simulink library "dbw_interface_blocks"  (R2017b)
settings: Solver=ode1  StartTime=0.0  StopTime=Inf  FixedStep=0.001  RelTol=1e-3  EnableMultiTasking=on
PostLoadFcn:
  | , if any(exist('dsrtsu_mdlpostloadfcn', 'file') == [2, 3, 6]), try dsrtsu_mdlpostloadfcn('Execute', bdroot); catch fprintf('Error in PostLoadFcn (dsrtsu_mdlpostloadfcn) for model "%s":\n %s\n', bdroot, lasterr); end, end,
libraries: rtican x9

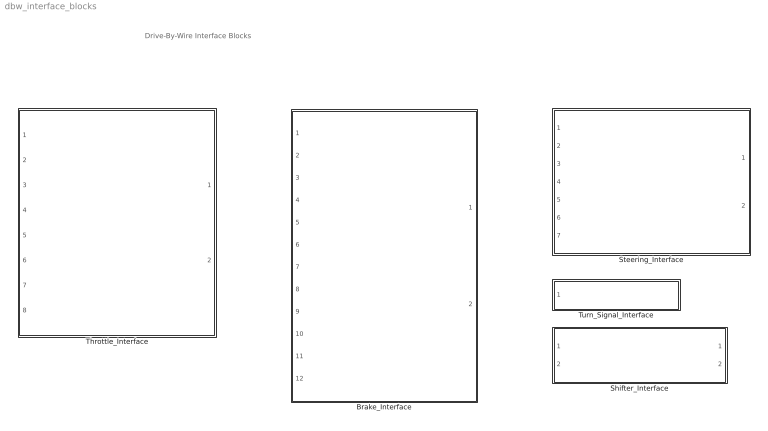
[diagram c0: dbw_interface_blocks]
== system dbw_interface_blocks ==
  note: Drive-By-Wire Interface Blocks
  Brake_Interface : Subsystem
  Shifter_Interface : Subsystem
  Steering_Interface : Subsystem
  Throttle_Interface : Subsystem
  Turn_Signal_Interface : Subsystem

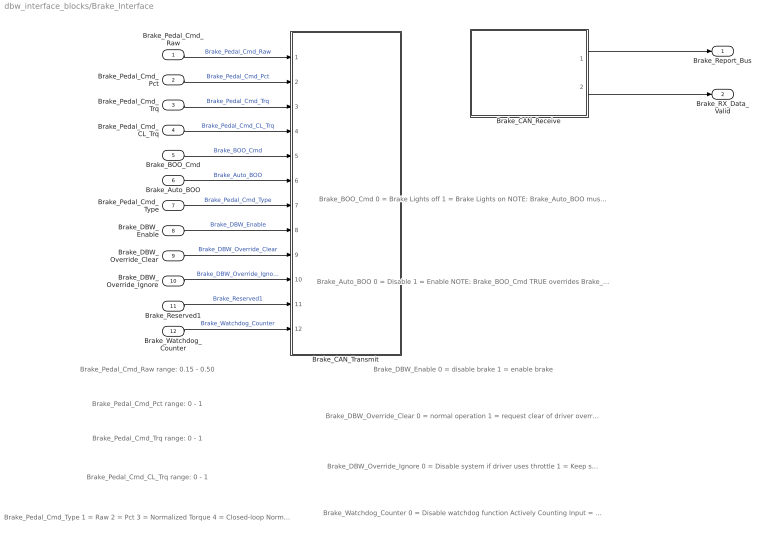
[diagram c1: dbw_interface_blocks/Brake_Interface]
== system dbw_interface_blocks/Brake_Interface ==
  note: Brake_Watchdog_Counter 0 = Disable watchdog function Actively Counting Input = Enable watchdog function
  note: Brake_DBW_Override_Ignore 0 = Disable system if driver uses throttle 1 = Keep system enabled if driver uses throttle
  note: Brake_DBW_Override_Clear 0 = normal operation 1 = request clear of driver override
  note: Brake_BOO_Cmd 0 = Brake Lights off 1 = Brake Lights on NOTE: Brake_Auto_BOO must be set to FALSE for user to have full control over Brake Lights On/Off.
  note: Brake_Pedal_Cmd_Raw range: 0.15 - 0.50
  note: Brake_DBW_Enable 0 = disable brake 1 = enable brake
  note: Brake_Pedal_Cmd_Pct range: 0 - 1
  note: Brake_Pedal_Cmd_Type 1 = Raw 2 = Pct 3 = Normalized Torque 4 = Closed-loop Normalized Torque
  note: Brake_Pedal_Cmd_Trq range: 0 - 1
  note: Brake_Pedal_Cmd_CL_Trq range: 0 - 1
  note: Brake_Auto_BOO 0 = Disable 1 = Enable NOTE: Brake_BOO_Cmd TRUE overrides Brake_Auto_BOO .
  Brake_Pedal_Cmd_Raw : Inport
  Brake_Pedal_Cmd_Pct : Inport  Port=2
  Brake_Pedal_Cmd_Trq : Inport  Port=3
  Brake_Pedal_Cmd_CL_Trq : Inport  Port=4
  Brake_BOO_Cmd : Inport  Port=5
  Brake_Auto_BOO : Inport  Port=6
  Brake_Pedal_Cmd_Type : Inport  Port=7
  Brake_DBW_Enable : Inport  Port=8
  Brake_DBW_Override_Clear : Inport  Port=9
  Brake_DBW_Override_Ignore : Inport  Port=10
  Brake_Reserved1 : Inport  Port=11
  Brake_Watchdog_Counter : Inport  Port=12
  Brake_CAN_Receive : Subsystem
  Brake_CAN_Transmit : Subsystem
  Brake_Report_Bus : Outport
  Brake_RX_Data_Valid : Outport  Port=2
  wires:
  Brake_Watchdog_Counter/1 -> Brake_CAN_Transmit/12(Brake_Watchdog_Counter)  "Brake_Watchdog_Counter"
  Brake_DBW_Override_Ignore/1 -> Brake_CAN_Transmit/10(Brake_DBW_Override_Ignore)  "Brake_DBW_Override_Ignore"
  Brake_CAN_Receive/1(Brake_Report_Bus) -> Brake_Report_Bus/1
  Brake_DBW_Override_Clear/1 -> Brake_CAN_Transmit/9(Brake_DBW_Override_Clear)  "Brake_DBW_Override_Clear"
  Brake_CAN_Receive/2(Brake_RX_Data_Valid) -> Brake_RX_Data_Valid/1
  Brake_BOO_Cmd/1 -> Brake_CAN_Transmit/5(Brake_BOO_Cmd)  "Brake_BOO_Cmd"
  Brake_DBW_Enable/1 -> Brake_CAN_Transmit/8(Brake_DBW_Enable)  "Brake_DBW_Enable"
  Brake_Reserved1/1 -> Brake_CAN_Transmit/11(Brake_Reserved1)  "Brake_Reserved1"
  Brake_Auto_BOO/1 -> Brake_CAN_Transmit/6(Brake_Auto_BOO)  "Brake_Auto_BOO"
  Brake_Pedal_Cmd_Type/1 -> Brake_CAN_Transmit/7(Brake_Pedal_Cmd_Type)  "Brake_Pedal_Cmd_Type"
  Brake_Pedal_Cmd_Pct/1 -> Brake_CAN_Transmit/2(Brake_Pedal_Cmd_Pct)  "Brake_Pedal_Cmd_Pct"
  Brake_Pedal_Cmd_Raw/1 -> Brake_CAN_Transmit/1(Brake_Pedal_Cmd_Raw)  "Brake_Pedal_Cmd_Raw"
  Brake_Pedal_Cmd_Trq/1 -> Brake_CAN_Transmit/3(Brake_Pedal_Cmd_Trq)  "Brake_Pedal_Cmd_Trq"
  Brake_Pedal_Cmd_CL_Trq/1 -> Brake_CAN_Transmit/4(Brake_Pedal_Cmd_CL_Trq)  "Brake_Pedal_Cmd_CL_Trq"

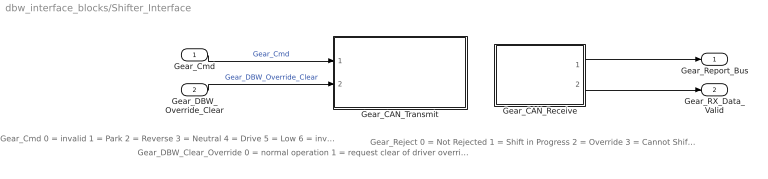
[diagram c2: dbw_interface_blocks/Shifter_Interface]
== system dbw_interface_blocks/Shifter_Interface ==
  note: Gear_DBW_Clear_Override 0 = normal operation 1 = request clear of driver override
  note: Gear_Cmd 0 = invalid 1 = Park 2 = Reverse 3 = Neutral 4 = Drive 5 = Low 6 = invalid 7 = invalid
  note: Gear_Reject 0 = Not Rejected 1 = Shift in Progress 2 = Override 3 = Cannot Shift to Low 4 = Cannot Shift out of Park 5 = Rejected (Brake not Pressed)
  Gear_Cmd : Inport
  Gear_DBW_Override_Clear : Inport  Port=2
  Gear_CAN_Receive : Subsystem
  Gear_CAN_Transmit : Subsystem
  Gear_Report_Bus : Outport
  Gear_RX_Data_Valid : Outport  Port=2
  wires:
  Gear_DBW_Override_Clear/1 -> Gear_CAN_Transmit/2(Gear_DBW_Override_Clear)  "Gear_DBW_Override_Clear"
  Gear_CAN_Receive/2(Gear_RX_Data_Valid) -> Gear_RX_Data_Valid/1
  Gear_CAN_Receive/1(Gear_Report_Bus) -> Gear_Report_Bus/1
  Gear_Cmd/1 -> Gear_CAN_Transmit/1(Gear_Cmd)  "Gear_Cmd"

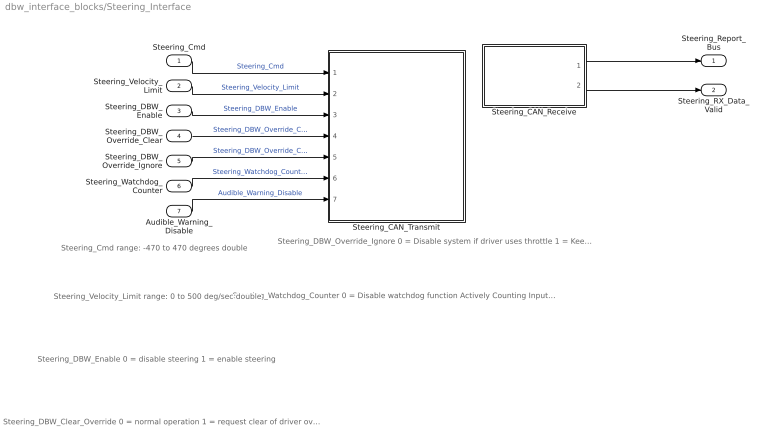
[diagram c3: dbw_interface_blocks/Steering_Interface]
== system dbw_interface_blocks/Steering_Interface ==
  note: Steering_Watchdog_Counter 0 = Disable watchdog function Actively Counting Input = Enable watchdog function
  note: Steering_DBW_Override_Ignore 0 = Disable system if driver uses throttle 1 = Keep system enabled if driver uses throttle
  note: Steering_Velocity_Limit range: 0 to 500 deg/sec double
  note: Steering_DBW_Clear_Override 0 = normal operation 1 = request clear of driver override
  note: Steering_DBW_Enable 0 = disable steering 1 = enable steering
  note: Steering_Cmd range: -470 to 470 degrees double
  Steering_Cmd : Inport
  Steering_Velocity_Limit : Inport  Port=2
  Steering_DBW_Enable : Inport  Port=3
  Steering_DBW_Override_Clear : Inport  Port=4
  Steering_DBW_Override_Ignore : Inport  Port=5
  Steering_Watchdog_Counter : Inport  Port=6
  Audible_Warning_Disable : Inport  Port=7
  Steering_CAN_Receive : Subsystem
  Steering_CAN_Transmit : Subsystem
  Steering_Report_Bus : Outport
  Steering_RX_Data_Valid : Outport  Port=2
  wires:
  Steering_Watchdog_Counter/1 -> Steering_CAN_Transmit/6(Steering_Watchdog_Counter)  "Steering_Watchdog_Counter"
  Steering_DBW_Override_Ignore/1 -> Steering_CAN_Transmit/5(Steering_DBW_Override_Ignore)  "Steering_DBW_Override_Clear"
  Steering_Velocity_Limit/1 -> Steering_CAN_Transmit/2(Steering_Velocity_Limit)  "Steering_Velocity_Limit"
  Steering_DBW_Override_Clear/1 -> Steering_CAN_Transmit/4(Steering_DBW_Clear_Override)  "Steering_DBW_Override_Clear"
  Steering_Cmd/1 -> Steering_CAN_Transmit/1(Steering_Cmd)  "Steering_Cmd"
  Steering_DBW_Enable/1 -> Steering_CAN_Transmit/3(Steering_DBW_Enable)  "Steering_DBW_Enable"
  Steering_CAN_Receive/1(Steering_Report_Bus) -> Steering_Report_Bus/1
  Steering_CAN_Receive/2(Steering_RX_Data_Valid) -> Steering_RX_Data_Valid/1
  Audible_Warning_Disable/1 -> Steering_CAN_Transmit/7(Audible_Warning_Disable)  "Audible_Warning_Disable"

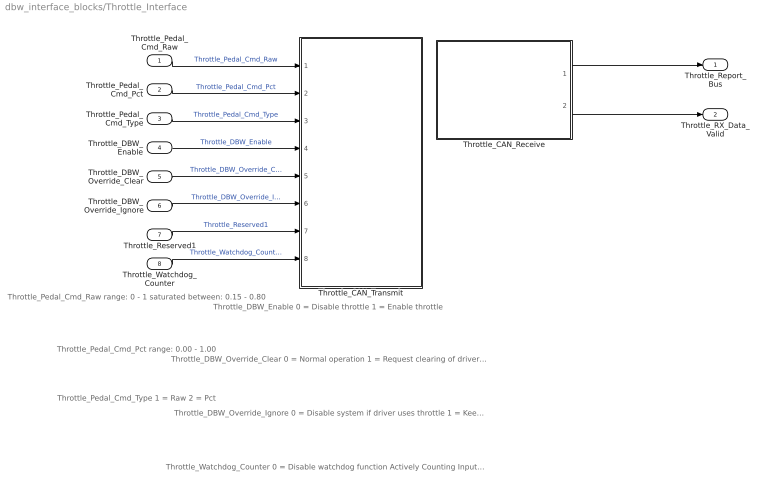
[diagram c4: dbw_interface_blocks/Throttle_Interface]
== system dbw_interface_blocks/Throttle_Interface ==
  note: Throttle_Watchdog_Counter 0 = Disable watchdog function Actively Counting Input = Enable watchdog function
  note: Throttle_DBW_Override_Clear 0 = Normal operation 1 = Request clearing of driver override
  note: Throttle_DBW_Enable 0 = Disable throttle 1 = Enable throttle
  note: Throttle_Pedal_Cmd_Raw range: 0 - 1 saturated between: 0.15 - 0.80
  note: Throttle_DBW_Override_Ignore 0 = Disable system if driver uses throttle 1 = Keep system enabled if driver uses throttle
  note: Throttle_Pedal_Cmd_Pct range: 0.00 - 1.00
  note: Throttle_Pedal_Cmd_Type 1 = Raw 2 = Pct
  Throttle_Pedal_Cmd_Raw : Inport
  Throttle_Pedal_Cmd_Pct : Inport  Port=2
  Throttle_Pedal_Cmd_Type : Inport  Port=3
  Throttle_DBW_Enable : Inport  Port=4
  Throttle_DBW_Override_Clear : Inport  Port=5
  Throttle_DBW_Override_Ignore : Inport  Port=6
  Throttle_Reserved1 : Inport  Port=7
  Throttle_Watchdog_Counter : Inport  Port=8
  Throttle_CAN_Receive : Subsystem
  Throttle_CAN_Transmit : Subsystem
  Throttle_Report_Bus : Outport
  Throttle_RX_Data_Valid : Outport  Port=2
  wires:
  Throttle_Watchdog_Counter/1 -> Throttle_CAN_Transmit/8(Throttle_Watchdog_Counter)  "Throttle_Watchdog_Counter"
  Throttle_DBW_Override_Ignore/1 -> Throttle_CAN_Transmit/6(Throttle_DBW_Override_Ignore)  "Throttle_DBW_Override_Ignore"
  Throttle_DBW_Override_Clear/1 -> Throttle_CAN_Transmit/5(Throttle_DBW_Override_Clear)  "Throttle_DBW_Override_Clear"
  Throttle_CAN_Receive/1(Throttle_Report_Bus) -> Throttle_Report_Bus/1
  Throttle_DBW_Enable/1 -> Throttle_CAN_Transmit/4(Throttle_DBW_Enable)  "Throttle_DBW_Enable"
  Throttle_CAN_Receive/2(Throttle_RX_Data_Valid) -> Throttle_RX_Data_Valid/1
  Throttle_Reserved1/1 -> Throttle_CAN_Transmit/7(Throttle_Reserved1)  "Throttle_Reserved1"
  Throttle_Pedal_Cmd_Raw/1 -> Throttle_CAN_Transmit/1(Throttle_Pedal_Cmd_Raw)  "Throttle_Pedal_Cmd_Raw"
  Throttle_Pedal_Cmd_Pct/1 -> Throttle_CAN_Transmit/2(Throttle_Pedal_Cmd_Pct)  "Throttle_Pedal_Cmd_Pct"
  Throttle_Pedal_Cmd_Type/1 -> Throttle_CAN_Transmit/3(Throttle_Pedal_Cmd_Type)  "Throttle_Pedal_Cmd_Type"

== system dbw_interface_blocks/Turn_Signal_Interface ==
  note: Turn_Signal_Cmd 0 = Off 1 = Left 2 = Right 3 = Invalid
  Turn_Signal_Cmd : Inport
  Turn_Signal_CAN_Transmit : Subsystem
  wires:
  Turn_Signal_Cmd/1 -> Turn_Signal_CAN_Transmit/1(Turn_Signal_Cmd)  "Turn_Signal_Cmd"

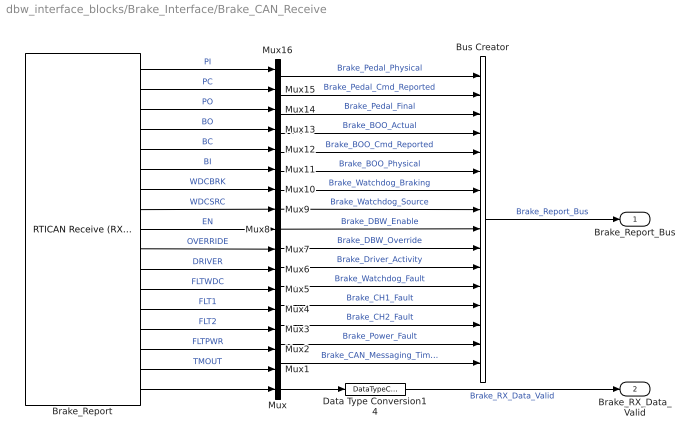
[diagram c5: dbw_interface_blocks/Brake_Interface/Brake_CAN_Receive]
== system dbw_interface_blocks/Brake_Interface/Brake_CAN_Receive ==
  Brake_Report : rtican/RTICAN Receive (RX)   Reserved1=[]  Reserved2=[]  Reserved3=[]  Reserved4=[]  SfcnMessage=[]  Msg_Struct=[]  BoardTypeNo=[]  BoardNo=[]  ChannelNo=[]  Parameters=[]  DialogFcn=[]  UnitName=[]  Revision=[]  UnitValues=[]  DSProperties=struct('RTI',struct('Version',uint32(5),'BlockType',struct('isSLSource',uint8(1),'isSLSink',uint8(1),'isHWSource',uint8(0),'isHWSink',uint8(0),'isSetup',uint8(0),'isInline',uint8(1),'isNonInline',uint8(0),'isInterrupt',uint8(0),'isChannelwise',uint8(0)),'IOBoardType','RTICAN','UnitType','MESSAGE','Identifier','RX','DialogType','MSVC','BlockSet','RTICAN','SlaveProcessor','CAN'))  RTIBlockInterface=struct('OutputPortsWidth',int32([1 1 1 1 1 1 1 1 1 1 1 1 1 1 1 1 1]),'OutputPortsActive',ones(1,17),'OutputPortsName',{{'PI','PC','PO','BO','BC','BI','WDCBRK','WDCSRC','EN','OVERRIDE','DRIVER','FLTWDC','FLT1','FLT2','FLTPWR','TMOUT',['RX status']}},'OutputPortsDataType',{{'SS_DOUBLE','SS_DOUBLE','SS_DOUBLE','SS_BOOLEAN','SS_BOOLEAN','SS_BOOLEAN','SS_BOOLEAN','SS_UINT8','SS_BOOLEAN','SS_BOOLEAN','S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  RTIBlockParameters=struct('BoardTypeNo',{{1,'OFF',[]}},'BoardNo',{{1,'ON',[1 16]}},'ChannelNo',{{1,'ON',[1 2]}},'Parameters',{{struct('DataFileSupport',struct('DataFileSelectedMaster',1,'DataFileSelectedLocal',1,'DataFileName','c:\users\dataspeed\documents\matlab\dataspeed_dbw_dspace_simulink_library\lib\dataspeedbywire_19_oct_2017.dbc|','DataFileDate',['11-Jul-2018 12:27:42'],'SelectedFile','dataspeedbywire.dbc','I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  RTISFcnParameters=struct('SFcnRTICANMessage','struct','TLCFileName','char')  RTIBlockParaDefault=struct('BoardTypeNo',4302,'BoardNo',1,'ChannelNo',1,'Parameters',struct('DataFileSupport',struct('DataFileSelectedMaster',0,'DataFileSelectedLocal',0,'DataFileName','','DataFileDate','','SelectedFile',['<no file selected>']),'Options',struct('StatusSelected',1,'TimeSelected',1,'DeltaTimeSelected',1,'BytePortSelected',0,'MessageLengthSelected',0,'TriggerPort',struct('Selected',0,'TriggerType','risi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
  Bus Creator : BusCreator  Inputs=16
  Data Type Conversion14 : DataTypeConversion  OutDataTypeStr=boolean
  Mux{,1..16} (17 alike) : Mux  Inputs=1
  Brake_Report_Bus : Outport
  Brake_RX_Data_Valid : Outport  Port=2
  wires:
  Data Type Conversion14/1 -> Brake_RX_Data_Valid/1  "Brake_RX_Data_Valid"
  Mux13/1 -> Bus Creator/4  "Brake_BOO_Actual"
  Mux12/1 -> Bus Creator/5  "Brake_BOO_Cmd_Reported"
  Mux11/1 -> Bus Creator/6  "Brake_BOO_Physical"
  Mux10/1 -> Bus Creator/7  "Brake_Watchdog_Braking"
  Mux9/1 -> Bus Creator/8  "Brake_Watchdog_Source"
  Mux/1 -> Data Type Conversion14/1
  Mux8/1 -> Bus Creator/9  "Brake_DBW_Enable"
  Mux7/1 -> Bus Creator/10  "Brake_DBW_Override"
  Mux6/1 -> Bus Creator/11  "Brake_Driver_Activity"
  Mux5/1 -> Bus Creator/12  "Brake_Watchdog_Fault"
  Mux4/1 -> Bus Creator/13  "Brake_CH1_Fault"
  Mux3/1 -> Bus Creator/14  "Brake_CH2_Fault"
  Mux2/1 -> Bus Creator/15  "Brake_Power_Fault"
  Mux1/1 -> Bus Creator/16  "Brake_CAN_Messaging_Timeout"
  Mux14/1 -> Bus Creator/3  "Brake_Pedal_Final"
  Mux15/1 -> Bus Creator/2  "Brake_Pedal_Cmd_Reported"
  Mux16/1 -> Bus Creator/1  "Brake_Pedal_Physical"
  Brake_Report/17 -> Mux/1
  Brake_Report/14 -> Mux3/1  "FLT2"
  Brake_Report/13 -> Mux4/1  "FLT1"
  Brake_Report/12 -> Mux5/1  "FLTWDC"
  Brake_Report/11 -> Mux6/1  "DRIVER"
  Brake_Report/10 -> Mux7/1  "OVERRIDE"
  Brake_Report/9 -> Mux8/1  "EN"
  Brake_Report/8 -> Mux9/1  "WDCSRC"
  Brake_Report/7 -> Mux10/1  "WDCBRK"
  Brake_Report/6 -> Mux11/1  "BI"
  Brake_Report/5 -> Mux12/1  "BC"
  Brake_Report/4 -> Mux13/1  "BO"
  Brake_Report/3 -> Mux14/1  "PO"
  Brake_Report/2 -> Mux15/1  "PC"
  Brake_Report/1 -> Mux16/1  "PI"
  Bus Creator/1 -> Brake_Report_Bus/1  "Brake_Report_Bus"
  Brake_Report/16 -> Mux1/1  "TMOUT"
  Brake_Report/15 -> Mux2/1  "FLTPWR"

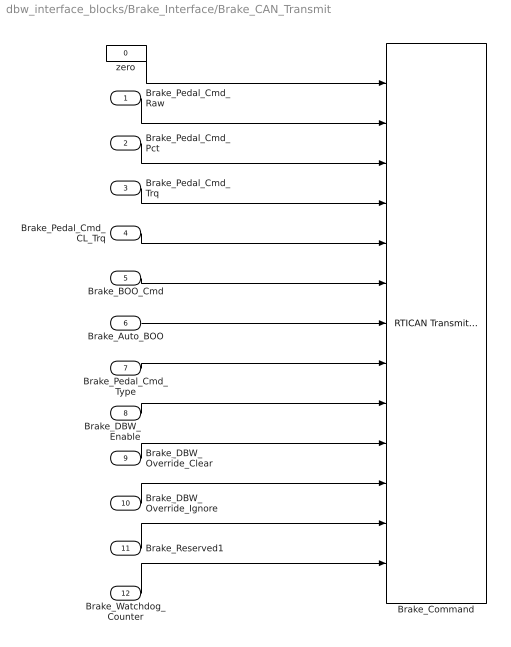
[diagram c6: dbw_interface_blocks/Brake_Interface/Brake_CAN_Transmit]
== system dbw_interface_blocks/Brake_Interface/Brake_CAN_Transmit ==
  Brake_Pedal_Cmd_Raw : Inport
  Brake_Pedal_Cmd_Pct : Inport  Port=2
  Brake_Pedal_Cmd_Trq : Inport  Port=3
  Brake_Pedal_Cmd_CL_Trq : Inport  Port=4
  Brake_BOO_Cmd : Inport  Port=5
  Brake_Auto_BOO : Inport  Port=6
  Brake_Pedal_Cmd_Type : Inport  Port=7
  Brake_DBW_Enable : Inport  Port=8
  Brake_DBW_Override_Clear : Inport  Port=9
  Brake_DBW_Override_Ignore : Inport  Port=10
  Brake_Reserved1 : Inport  Port=11
  Brake_Watchdog_Counter : Inport  Port=12
  Brake_Command : rtican/RTICAN Transmit (TX)   Reserved1=[]  Reserved2=[]  Reserved3=[]  Reserved4=[]  SfcnMessage=[]  Msg_Struct=[]  BoardTypeNo=[]  BoardNo=[]  ChannelNo=[]  Parameters=[]  DialogFcn=[]  UnitName=[]  Revision=[]  UnitValues=[]  DSProperties=struct('RTI',struct('Version',uint32(5),'BlockType',struct('isSLSource',uint8(1),'isSLSink',uint8(1),'isHWSource',uint8(0),'isHWSink',uint8(0),'isSetup',uint8(0),'isInline',uint8(1),'isNonInline',uint8(0),'isInterrupt',uint8(0),'isChannelwise',uint8(0)),'IOBoardType','RTICAN','UnitType','MESSAGE','Identifier','TX','DialogType','MSVC','BlockSet','RTICAN','SlaveProcessor','CAN'))  RTIBlockInterface=struct('InputPortsWidth',int32([1 1 1 1 1 1 1 1 1 1 1 1 1]),'InputPortsActive',ones(1,13),'InputPortsName',{{'PCMD_NONE','PCMD_PEDAL','PCMD_PERCENT','PCMD_TORQUE','PCMD_TORQUE_RQ','BCMD','ABOO','CMD_TYPE','EN','CLEAR','IGNORE','RES1','COUNT'}},'InputPortsDataType',{{'SS_DOUBLE','SS_DOUBLE','SS_DOUBLE','SS_UINT16','SS_UINT16','SS_BOOLEAN','SS_BOOLEAN','SS_UINT8','SS_BOOLEAN','SS_BOOLEAN','SS_BOOLEA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  RTIBlockParameters=struct('BoardTypeNo',{{1,'OFF',[]}},'BoardNo',{{1,'ON',[1 16]}},'ChannelNo',{{1,'ON',[1 2]}},'Parameters',{{struct('DataFileSupport',struct('DataFileSelectedMaster',1,'DataFileSelectedLocal',1,'DataFileName','c:\users\dataspeed\documents\matlab\dataspeed_dbw_dspace_simulink_library\lib\dataspeedbywire_19_oct_2017.dbc|','DataFileDate',['11-Jul-2018 12:27:42'],'SelectedFile','dataspeedbywire.dbc','I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  RTISFcnParameters=struct('SFcnRTICANMessage','struct','TLCFileName','char')  RTIBlockParaDefault=struct('BoardTypeNo',4302,'BoardNo',1,'ChannelNo',1,'Parameters',struct('DataFileSupport',struct('DataFileSelectedMaster',0,'DataFileSelectedLocal',0,'DataFileName','','DataFileDate','','SelectedFile',['<no file selected>']),'Options',struct('StatusSelected',1,'TimeSelected',1,'DeltaTimeSelected',1,'DelayTimeSelected',1,'DelayTimeTXCommandSelected',0,'EncodeSetUnusedBitsToOne',0,'EnableMsgLoopback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
  zero : Constant  Value=0
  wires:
  Brake_DBW_Enable/1 -> Brake_Command/9
  Brake_DBW_Override_Clear/1 -> Brake_Command/10
  Brake_DBW_Override_Ignore/1 -> Brake_Command/11
  Brake_Watchdog_Counter/1 -> Brake_Command/13
  Brake_Reserved1/1 -> Brake_Command/12
  Brake_BOO_Cmd/1 -> Brake_Command/6
  Brake_Auto_BOO/1 -> Brake_Command/7
  Brake_Pedal_Cmd_Type/1 -> Brake_Command/8
  Brake_Pedal_Cmd_Trq/1 -> Brake_Command/4
  Brake_Pedal_Cmd_Pct/1 -> Brake_Command/3
  Brake_Pedal_Cmd_Raw/1 -> Brake_Command/2
  Brake_Pedal_Cmd_CL_Trq/1 -> Brake_Command/5
  zero/1 -> Brake_Command/1

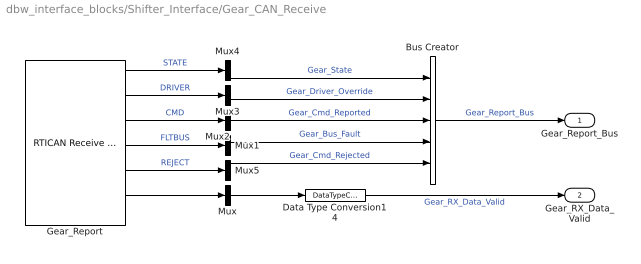
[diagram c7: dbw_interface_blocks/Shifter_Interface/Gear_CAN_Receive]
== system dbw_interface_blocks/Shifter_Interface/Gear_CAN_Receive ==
  Bus Creator : BusCreator  Inputs=5
  Data Type Conversion14 : DataTypeConversion  OutDataTypeStr=boolean
  Gear_Report : rtican/RTICAN Receive (RX)   Reserved1=[]  Reserved2=[]  Reserved3=[]  Reserved4=[]  SfcnMessage=[]  Msg_Struct=[]  BoardTypeNo=[]  BoardNo=[]  ChannelNo=[]  Parameters=[]  DialogFcn=[]  UnitName=[]  Revision=[]  UnitValues=[]  DSProperties=struct('RTI',struct('Version',uint32(5),'BlockType',struct('isSLSource',uint8(1),'isSLSink',uint8(1),'isHWSource',uint8(0),'isHWSink',uint8(0),'isSetup',uint8(0),'isInline',uint8(1),'isNonInline',uint8(0),'isInterrupt',uint8(0),'isChannelwise',uint8(0)),'IOBoardType','RTICAN','UnitType','MESSAGE','Identifier','RX','DialogType','MSVC','BlockSet','RTICAN','SlaveProcessor','CAN'))  RTIBlockInterface=struct('OutputPortsWidth',int32([1 1 1 1 1 1]),'OutputPortsActive',[1 1 1 1 1 1],'OutputPortsName',{{'STATE','DRIVER','CMD','FLTBUS','REJECT',['RX status']}},'OutputPortsDataType',{{'SS_UINT8','SS_BOOLEAN','SS_UINT8','SS_BOOLEAN','SS_UINT8','SS_DOUBLE'}},'OutputPortsLabel',{{'STATE','DRIVER','CMD','FLTBUS','REJECT',''}},'OutputPortsLabelMode','ON','InputPortsWidth',int32(0),'InputPortsActive',0,'D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  RTIBlockParameters=struct('BoardTypeNo',{{1,'OFF',[]}},'BoardNo',{{1,'ON',[1 16]}},'ChannelNo',{{1,'ON',[1 2]}},'Parameters',{{struct('DataFileSupport',struct('DataFileSelectedMaster',1,'DataFileSelectedLocal',1,'DataFileName','c:\users\dataspeed\documents\matlab\dataspeed_dbw_dspace_simulink_library\lib\dataspeedbywire_19_oct_2017.dbc|','DataFileDate',['11-Jul-2018 12:27:42'],'SelectedFile','dataspeedbywire.dbc','I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  RTISFcnParameters=struct('SFcnRTICANMessage','struct','TLCFileName','char')  RTIBlockParaDefault=struct('BoardTypeNo',4302,'BoardNo',1,'ChannelNo',1,'Parameters',struct('DataFileSupport',struct('DataFileSelectedMaster',0,'DataFileSelectedLocal',0,'DataFileName','','DataFileDate','','SelectedFile',['<no file selected>']),'Options',struct('StatusSelected',1,'TimeSelected',1,'DeltaTimeSelected',1,'BytePortSelected',0,'MessageLengthSelected',0,'TriggerPort',struct('Selected',0,'TriggerType','risi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
  Mux{,1..5} (6 alike) : Mux  Inputs=1
  Gear_Report_Bus : Outport
  Gear_RX_Data_Valid : Outport  Port=2
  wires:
  Data Type Conversion14/1 -> Gear_RX_Data_Valid/1  "Gear_RX_Data_Valid"
  Mux/1 -> Data Type Conversion14/1
  Mux1/1 -> Bus Creator/4  "Gear_Bus_Fault"
  Mux2/1 -> Bus Creator/3  "Gear_Cmd_Reported"
  Mux3/1 -> Bus Creator/2  "Gear_Driver_Override"
  Mux4/1 -> Bus Creator/1  "Gear_State"
  Gear_Report/6 -> Mux/1
  Gear_Report/4 -> Mux1/1  "FLTBUS"
  Gear_Report/3 -> Mux2/1  "CMD"
  Gear_Report/2 -> Mux3/1  "DRIVER"
  Gear_Report/1 -> Mux4/1  "STATE"
  Bus Creator/1 -> Gear_Report_Bus/1  "Gear_Report_Bus"
  Gear_Report/5 -> Mux5/1  "REJECT"
  Mux5/1 -> Bus Creator/5  "Gear_Cmd_Rejected"

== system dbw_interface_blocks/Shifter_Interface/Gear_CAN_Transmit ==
  Gear_Cmd : Inport
  Gear_DBW_Override_Clear : Inport  Port=2
  Data Type Conversion : DataTypeConversion  OutDataTypeStr=uint8
  Gear_Command1 : rtican/RTICAN Transmit (TX)   Reserved1=[]  Reserved2=[]  Reserved3=[]  Reserved4=[]  SfcnMessage=[]  Msg_Struct=[]  BoardTypeNo=[]  BoardNo=[]  ChannelNo=[]  Parameters=[]  DialogFcn=[]  UnitName=[]  Revision=[]  UnitValues=[]  DSProperties=struct('RTI',struct('Version',uint32(5),'BlockType',struct('isSLSource',uint8(1),'isSLSink',uint8(1),'isHWSource',uint8(0),'isHWSink',uint8(0),'isSetup',uint8(0),'isInline',uint8(1),'isNonInline',uint8(0),'isInterrupt',uint8(0),'isChannelwise',uint8(0)),'IOBoardType','RTICAN','UnitType','MESSAGE','Identifier','TX','DialogType','MSVC','BlockSet','RTICAN','SlaveProcessor','CAN'))  RTIBlockInterface=struct('InputPortsWidth',int32([1 1]),'InputPortsActive',[1 1],'InputPortsName',{{'GCMD','CLEAR'}},'InputPortsDataType',{{'SS_UINT8','SS_BOOLEAN'}},'OutputPortsWidth',int32(0),'OutputPortsActive',0,'OutputPortsName',{{''}},'DialogFcn','rtican_message_interface_gui','BlockDisplay',{{'','center'}},'IconTransparency','on','InitLevel',3,'BlockName',struct('Token',{{'Gear_Command'}}),'SampleTime',{{0.1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  RTIBlockParameters=struct('BoardTypeNo',{{1,'OFF',[]}},'BoardNo',{{1,'ON',[1 16]}},'ChannelNo',{{1,'ON',[1 2]}},'Parameters',{{struct('DataFileSupport',struct('DataFileSelectedMaster',1,'DataFileSelectedLocal',1,'DataFileName','c:\users\dataspeed\documents\matlab\dataspeed_dbw_dspace_simulink_library\lib\dataspeedbywire_19_oct_2017.dbc|','DataFileDate',['11-Jul-2018 12:27:42'],'SelectedFile','dataspeedbywire.dbc','I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  RTISFcnParameters=struct('SFcnRTICANMessage','struct','TLCFileName','char')  RTIBlockParaDefault=struct('BoardTypeNo',4302,'BoardNo',1,'ChannelNo',1,'Parameters',struct('DataFileSupport',struct('DataFileSelectedMaster',0,'DataFileSelectedLocal',0,'DataFileName','','DataFileDate','','SelectedFile',['<no file selected>']),'Options',struct('StatusSelected',1,'TimeSelected',1,'DeltaTimeSelected',1,'DelayTimeSelected',1,'DelayTimeTXCommandSelected',0,'EncodeSetUnusedBitsToOne',0,'EnableMsgLoopback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
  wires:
  Gear_DBW_Override_Clear/1 -> Gear_Command1/2  "Gear_DBW_Override_Clear"
  Data Type Conversion/1 -> Gear_Command1/1
  Gear_Cmd/1 -> Data Type Conversion/1  "Gear_Cmd"

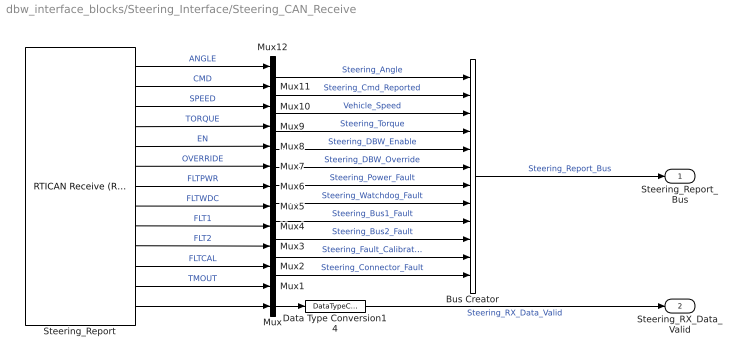
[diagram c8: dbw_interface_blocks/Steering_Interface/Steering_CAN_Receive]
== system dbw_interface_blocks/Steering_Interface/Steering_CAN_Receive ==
  Bus Creator : BusCreator  Inputs=12
  Data Type Conversion14 : DataTypeConversion  OutDataTypeStr=boolean
  Mux{,1..12} (13 alike) : Mux  Inputs=1
  Steering_Report : rtican/RTICAN Receive (RX)   Reserved1=[]  Reserved2=[]  Reserved3=[]  Reserved4=[]  SfcnMessage=[]  Msg_Struct=[]  BoardTypeNo=[]  BoardNo=[]  ChannelNo=[]  Parameters=[]  DialogFcn=[]  UnitName=[]  Revision=[]  UnitValues=[]  DSProperties=struct('RTI',struct('Version',uint32(5),'BlockType',struct('isSLSource',uint8(1),'isSLSink',uint8(1),'isHWSource',uint8(0),'isHWSink',uint8(0),'isSetup',uint8(0),'isInline',uint8(1),'isNonInline',uint8(0),'isInterrupt',uint8(0),'isChannelwise',uint8(0)),'IOBoardType','RTICAN','UnitType','MESSAGE','Identifier','RX','DialogType','MSVC','BlockSet','RTICAN','SlaveProcessor','CAN'))  RTIBlockInterface=struct('OutputPortsWidth',int32([1 1 1 1 1 1 1 1 1 1 1 1 1]),'OutputPortsActive',ones(1,13),'OutputPortsName',{{'ANGLE','CMD','SPEED','TORQUE','EN','OVERRIDE','FLTPWR','FLTWDC','FLT1','FLT2','FLTCAL','TMOUT',['RX status']}},'OutputPortsDataType',{{'SS_DOUBLE','SS_DOUBLE','SS_DOUBLE','SS_DOUBLE','SS_BOOLEAN','SS_BOOLEAN','SS_BOOLEAN','SS_BOOLEAN','SS_BOOLEAN','SS_BOOLEAN','SS_BOOLEAN','SS_BOOLEAN',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  RTIBlockParameters=struct('BoardTypeNo',{{1,'OFF',[]}},'BoardNo',{{1,'ON',[1 16]}},'ChannelNo',{{1,'ON',[1 2]}},'Parameters',{{struct('DataFileSupport',struct('DataFileSelectedMaster',1,'DataFileSelectedLocal',1,'DataFileName','c:\users\dataspeed\documents\matlab\dataspeed_dbw_dspace_simulink_library\lib\dataspeedbywire_19_oct_2017.dbc|','DataFileDate',['11-Jul-2018 12:27:42'],'SelectedFile','dataspeedbywire.dbc','I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  RTISFcnParameters=struct('SFcnRTICANMessage','struct','TLCFileName','char')  RTIBlockParaDefault=struct('BoardTypeNo',4302,'BoardNo',1,'ChannelNo',1,'Parameters',struct('DataFileSupport',struct('DataFileSelectedMaster',0,'DataFileSelectedLocal',0,'DataFileName','','DataFileDate','','SelectedFile',['<no file selected>']),'Options',struct('StatusSelected',1,'TimeSelected',1,'DeltaTimeSelected',1,'BytePortSelected',0,'MessageLengthSelected',0,'TriggerPort',struct('Selected',0,'TriggerType','risi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
  Steering_Report_Bus : Outport
  Steering_RX_Data_Valid : Outport  Port=2
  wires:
  Mux8/1 -> Bus Creator/5  "Steering_DBW_Enable"
  Mux7/1 -> Bus Creator/6  "Steering_DBW_Override"
  Mux5/1 -> Bus Creator/8  "Steering_Watchdog_Fault"
  Mux4/1 -> Bus Creator/9  "Steering_Bus1_Fault"
  Mux3/1 -> Bus Creator/10  "Steering_Bus2_Fault"
  Mux2/1 -> Bus Creator/11  "Steering_Fault_Calibration"
  Mux1/1 -> Bus Creator/12  "Steering_Connector_Fault"
  Data Type Conversion14/1 -> Steering_RX_Data_Valid/1  "Steering_RX_Data_Valid"
  Mux/1 -> Data Type Conversion14/1
  Mux9/1 -> Bus Creator/4  "Steering_Torque"
  Mux10/1 -> Bus Creator/3  "Vehicle_Speed"
  Mux11/1 -> Bus Creator/2  "Steering_Cmd_Reported"
  Mux12/1 -> Bus Creator/1  "Steering_Angle"
  Steering_Report/11 -> Mux2/1  "FLTCAL"
  Steering_Report/10 -> Mux3/1  "FLT2"
  Steering_Report/9 -> Mux4/1  "FLT1"
  Steering_Report/8 -> Mux5/1  "FLTWDC"
  Steering_Report/6 -> Mux7/1  "OVERRIDE"
  Steering_Report/5 -> Mux8/1  "EN"
  Steering_Report/4 -> Mux9/1  "TORQUE"
  Steering_Report/3 -> Mux10/1  "SPEED"
  Steering_Report/2 -> Mux11/1  "CMD"
  Steering_Report/1 -> Mux12/1  "ANGLE"
  Bus Creator/1 -> Steering_Report_Bus/1  "Steering_Report_Bus"
  Steering_Report/12 -> Mux1/1  "TMOUT"
  Steering_Report/7 -> Mux6/1  "FLTPWR"
  Mux6/1 -> Bus Creator/7  "Steering_Power_Fault"
  Steering_Report/13 -> Mux/1

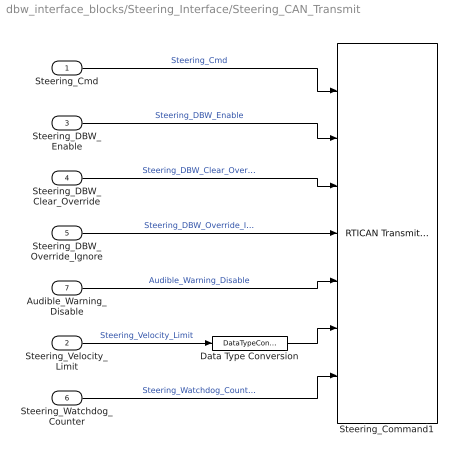
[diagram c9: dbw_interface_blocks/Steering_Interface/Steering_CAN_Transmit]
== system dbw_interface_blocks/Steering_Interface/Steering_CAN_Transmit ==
  Steering_Cmd : Inport
  Steering_Velocity_Limit : Inport  Port=2
  Steering_DBW_Enable : Inport  Port=3
  Steering_DBW_Clear_Override : Inport  Port=4
  Steering_DBW_Override_Ignore : Inport  Port=5
  Steering_Watchdog_Counter : Inport  Port=6
  Audible_Warning_Disable : Inport  Port=7
  Data Type Conversion : DataTypeConversion
  Steering_Command1 : rtican/RTICAN Transmit (TX)   Reserved1=[]  Reserved2=[]  Reserved3=[]  Reserved4=[]  SfcnMessage=[]  Msg_Struct=[]  BoardTypeNo=[]  BoardNo=[]  ChannelNo=[]  Parameters=[]  DialogFcn=[]  UnitName=[]  Revision=[]  UnitValues=[]  DSProperties=struct('RTI',struct('Version',uint32(5),'BlockType',struct('isSLSource',uint8(1),'isSLSink',uint8(1),'isHWSource',uint8(0),'isHWSink',uint8(0),'isSetup',uint8(0),'isInline',uint8(1),'isNonInline',uint8(0),'isInterrupt',uint8(0),'isChannelwise',uint8(0)),'IOBoardType','RTICAN','UnitType','MESSAGE','Identifier','TX','DialogType','MSVC','BlockSet','RTICAN','SlaveProcessor','CAN'))  RTIBlockInterface=struct('InputPortsWidth',int32([1 1 1 1 1 1 1]),'InputPortsActive',[1 1 1 1 1 1 1],'InputPortsName',{{'SCMD','EN','CLEAR','IGNORE','QUIET','SVEL','COUNT'}},'InputPortsDataType',{{'SS_DOUBLE','SS_BOOLEAN','SS_BOOLEAN','SS_BOOLEAN','SS_BOOLEAN','SS_UINT16','SS_UINT8'}},'OutputPortsWidth',int32(0),'OutputPortsActive',0,'OutputPortsName',{{''}},'DialogFcn','rtican_message_interface_gui','BlockDisplay'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  RTIBlockParameters=struct('BoardTypeNo',{{1,'OFF',[]}},'BoardNo',{{1,'ON',[1 16]}},'ChannelNo',{{1,'ON',[1 2]}},'Parameters',{{struct('DataFileSupport',struct('DataFileSelectedMaster',1,'DataFileSelectedLocal',1,'DataFileName','c:\users\dataspeed\documents\matlab\dataspeed_dbw_dspace_simulink_library\lib\dataspeedbywire_19_oct_2017.dbc|','DataFileDate',['11-Jul-2018 12:27:42'],'SelectedFile','dataspeedbywire.dbc','I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  RTISFcnParameters=struct('SFcnRTICANMessage','struct','TLCFileName','char')  RTIBlockParaDefault=struct('BoardTypeNo',4302,'BoardNo',1,'ChannelNo',1,'Parameters',struct('DataFileSupport',struct('DataFileSelectedMaster',0,'DataFileSelectedLocal',0,'DataFileName','','DataFileDate','','SelectedFile',['<no file selected>']),'Options',struct('StatusSelected',1,'TimeSelected',1,'DeltaTimeSelected',1,'DelayTimeSelected',1,'DelayTimeTXCommandSelected',0,'EncodeSetUnusedBitsToOne',0,'EnableMsgLoopback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
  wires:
  Steering_Watchdog_Counter/1 -> Steering_Command1/7  "Steering_Watchdog_Counter"
  Steering_DBW_Override_Ignore/1 -> Steering_Command1/4  "Steering_DBW_Override_Ignore"
  Steering_Velocity_Limit/1 -> Data Type Conversion/1  "Steering_Velocity_Limit"
  Steering_DBW_Clear_Override/1 -> Steering_Command1/3  "Steering_DBW_Clear_Override"
  Steering_DBW_Enable/1 -> Steering_Command1/2  "Steering_DBW_Enable"
  Steering_Cmd/1 -> Steering_Command1/1  "Steering_Cmd"
  Data Type Conversion/1 -> Steering_Command1/6
  Audible_Warning_Disable/1 -> Steering_Command1/5  "Audible_Warning_Disable"

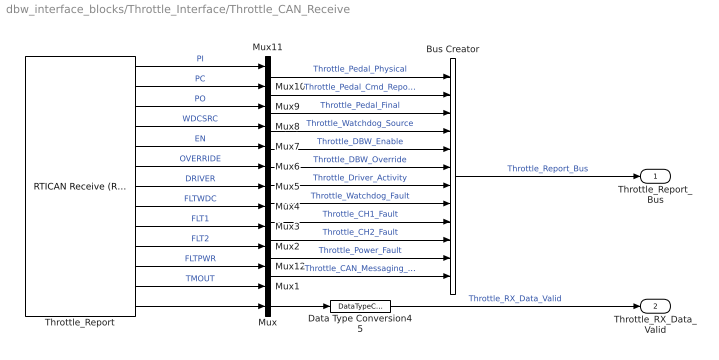
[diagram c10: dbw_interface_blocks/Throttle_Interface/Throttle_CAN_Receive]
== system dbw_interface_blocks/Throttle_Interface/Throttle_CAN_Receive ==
  Bus Creator : BusCreator  Inputs=12
  Data Type Conversion45 : DataTypeConversion  OutDataTypeStr=boolean
  Mux{,1..12} (13 alike) : Mux  Inputs=1
  Throttle_Report : rtican/RTICAN Receive (RX)   Reserved1=[]  Reserved2=[]  Reserved3=[]  Reserved4=[]  SfcnMessage=[]  Msg_Struct=[]  BoardTypeNo=[]  BoardNo=[]  ChannelNo=[]  Parameters=[]  DialogFcn=[]  UnitName=[]  Revision=[]  UnitValues=[]  DSProperties=struct('RTI',struct('Version',uint32(5),'BlockType',struct('isSLSource',uint8(1),'isSLSink',uint8(1),'isHWSource',uint8(0),'isHWSink',uint8(0),'isSetup',uint8(0),'isInline',uint8(1),'isNonInline',uint8(0),'isInterrupt',uint8(0),'isChannelwise',uint8(0)),'IOBoardType','RTICAN','UnitType','MESSAGE','Identifier','RX','DialogType','MSVC','BlockSet','RTICAN','SlaveProcessor','CAN'))  RTIBlockInterface=struct('OutputPortsWidth',int32([1 1 1 1 1 1 1 1 1 1 1 1 1]),'OutputPortsActive',ones(1,13),'OutputPortsName',{{'PI','PC','PO','WDCSRC','EN','OVERRIDE','DRIVER','FLTWDC','FLT1','FLT2','FLTPWR','TMOUT',['RX status']}},'OutputPortsDataType',{{'SS_DOUBLE','SS_DOUBLE','SS_DOUBLE','SS_UINT8','SS_BOOLEAN','SS_BOOLEAN','SS_BOOLEAN','SS_BOOLEAN','SS_BOOLEAN','SS_BOOLEAN','SS_BOOLEAN','SS_BOOLEAN','SS_DOUB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  RTIBlockParameters=struct('BoardTypeNo',{{1,'OFF',[]}},'BoardNo',{{1,'ON',[1 16]}},'ChannelNo',{{1,'ON',[1 2]}},'Parameters',{{struct('DataFileSupport',struct('DataFileSelectedMaster',1,'DataFileSelectedLocal',1,'DataFileName','c:\users\dataspeed\documents\matlab\dataspeed_dbw_dspace_simulink_library\lib\dataspeedbywire_19_oct_2017.dbc|','DataFileDate',['11-Jul-2018 12:27:42'],'SelectedFile','dataspeedbywire.dbc','I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  RTISFcnParameters=struct('SFcnRTICANMessage','struct','TLCFileName','char')  RTIBlockParaDefault=struct('BoardTypeNo',4302,'BoardNo',1,'ChannelNo',1,'Parameters',struct('DataFileSupport',struct('DataFileSelectedMaster',0,'DataFileSelectedLocal',0,'DataFileName','','DataFileDate','','SelectedFile',['<no file selected>']),'Options',struct('StatusSelected',1,'TimeSelected',1,'DeltaTimeSelected',1,'BytePortSelected',0,'MessageLengthSelected',0,'TriggerPort',struct('Selected',0,'TriggerType','risi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
  Throttle_Report_Bus : Outport
  Throttle_RX_Data_Valid : Outport  Port=2
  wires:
  Data Type Conversion45/1 -> Throttle_RX_Data_Valid/1  "Throttle_RX_Data_Valid"
  Mux8/1 -> Bus Creator/4  "Throttle_Watchdog_Source"
  Mux7/1 -> Bus Creator/5  "Throttle_DBW_Enable"
  Mux6/1 -> Bus Creator/6  "Throttle_DBW_Override"
  Mux5/1 -> Bus Creator/7  "Throttle_Driver_Activity"
  Mux4/1 -> Bus Creator/8  "Throttle_Watchdog_Fault"
  Mux3/1 -> Bus Creator/9  "Throttle_CH1_Fault"
  Mux2/1 -> Bus Creator/10  "Throttle_CH2_Fault"
  Mux1/1 -> Bus Creator/12  "Throttle_CAN_Messaging_Timeout"
  Mux/1 -> Data Type Conversion45/1
  Mux9/1 -> Bus Creator/3  "Throttle_Pedal_Final"
  Mux10/1 -> Bus Creator/2  "Throttle_Pedal_Cmd_Reported"
  Mux11/1 -> Bus Creator/1  "Throttle_Pedal_Physical"
  Throttle_Report/13 -> Mux/1
  Throttle_Report/10 -> Mux2/1  "FLT2"
  Throttle_Report/9 -> Mux3/1  "FLT1"
  Throttle_Report/8 -> Mux4/1  "FLTWDC"
  Throttle_Report/7 -> Mux5/1  "DRIVER"
  Throttle_Report/6 -> Mux6/1  "OVERRIDE"
  Throttle_Report/5 -> Mux7/1  "EN"
  Throttle_Report/4 -> Mux8/1  "WDCSRC"
  Throttle_Report/3 -> Mux9/1  "PO"
  Throttle_Report/2 -> Mux10/1  "PC"
  Throttle_Report/1 -> Mux11/1  "PI"
  Bus Creator/1 -> Throttle_Report_Bus/1  "Throttle_Report_Bus"
  Throttle_Report/12 -> Mux1/1  "TMOUT"
  Throttle_Report/11 -> Mux12/1  "FLTPWR"
  Mux12/1 -> Bus Creator/11  "Throttle_Power_Fault"

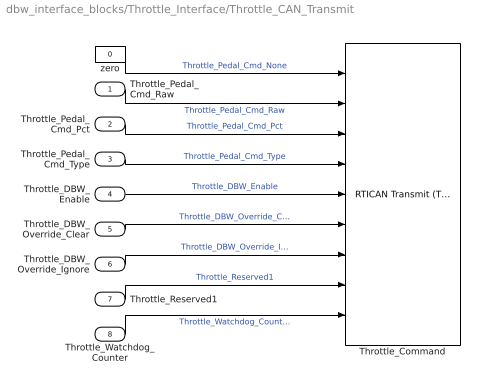
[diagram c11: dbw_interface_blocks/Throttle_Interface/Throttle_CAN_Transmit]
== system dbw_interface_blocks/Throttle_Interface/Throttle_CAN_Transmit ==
  Throttle_Pedal_Cmd_Raw : Inport
  Throttle_Pedal_Cmd_Pct : Inport  Port=2
  Throttle_Pedal_Cmd_Type : Inport  Port=3
  Throttle_DBW_Enable : Inport  Port=4
  Throttle_DBW_Override_Clear : Inport  Port=5
  Throttle_DBW_Override_Ignore : Inport  Port=6
  Throttle_Reserved1 : Inport  Port=7
  Throttle_Watchdog_Counter : Inport  Port=8
  Throttle_Command : rtican/RTICAN Transmit (TX)   Reserved1=[]  Reserved2=[]  Reserved3=[]  Reserved4=[]  SfcnMessage=[]  Msg_Struct=[]  BoardTypeNo=[]  BoardNo=[]  ChannelNo=[]  Parameters=[]  DialogFcn=[]  UnitName=[]  Revision=[]  UnitValues=[]  DSProperties=struct('RTI',struct('Version',uint32(5),'BlockType',struct('isSLSource',uint8(1),'isSLSink',uint8(1),'isHWSource',uint8(0),'isHWSink',uint8(0),'isSetup',uint8(0),'isInline',uint8(1),'isNonInline',uint8(0),'isInterrupt',uint8(0),'isChannelwise',uint8(0)),'IOBoardType','RTICAN','UnitType','MESSAGE','Identifier','TX','DialogType','MSVC','BlockSet','RTICAN','SlaveProcessor','CAN'))  RTIBlockInterface=struct('InputPortsWidth',int32([1 1 1 1 1 1 1 1 1]),'InputPortsActive',[1 1 1 1 1 1 1 1 1],'InputPortsName',{{'PCMD_NONE','PCMD_PEDAL','PCMD_PERCENT','CMD_TYPE','EN','CLEAR','IGNORE','RES1','COUNT'}},'InputPortsDataType',{{'SS_DOUBLE','SS_DOUBLE','SS_DOUBLE','SS_UINT8','SS_BOOLEAN','SS_BOOLEAN','SS_BOOLEAN','SS_BOOLEAN','SS_UINT8'}},'OutputPortsWidth',int32(0),'OutputPortsActive',0,'OutputPortsNam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  RTIBlockParameters=struct('BoardTypeNo',{{1,'OFF',[]}},'BoardNo',{{1,'ON',[1 16]}},'ChannelNo',{{1,'ON',[1 2]}},'Parameters',{{struct('DataFileSupport',struct('DataFileSelectedMaster',1,'DataFileSelectedLocal',1,'DataFileName','c:\users\dataspeed\documents\matlab\dataspeed_dbw_dspace_simulink_library\lib\dataspeedbywire_19_oct_2017.dbc|','DataFileDate',['11-Jul-2018 12:27:42'],'SelectedFile','dataspeedbywire.dbc','I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  RTISFcnParameters=struct('SFcnRTICANMessage','struct','TLCFileName','char')  RTIBlockParaDefault=struct('BoardTypeNo',4302,'BoardNo',1,'ChannelNo',1,'Parameters',struct('DataFileSupport',struct('DataFileSelectedMaster',0,'DataFileSelectedLocal',0,'DataFileName','','DataFileDate','','SelectedFile',['<no file selected>']),'Options',struct('StatusSelected',1,'TimeSelected',1,'DeltaTimeSelected',1,'DelayTimeSelected',1,'DelayTimeTXCommandSelected',0,'EncodeSetUnusedBitsToOne',0,'EnableMsgLoopback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
  zero : Constant  Value=0
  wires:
  Throttle_Watchdog_Counter/1 -> Throttle_Command/9  "Throttle_Watchdog_Counter"
  Throttle_DBW_Override_Ignore/1 -> Throttle_Command/7  "Throttle_DBW_Override_Ignore"
  Throttle_DBW_Override_Clear/1 -> Throttle_Command/6  "Throttle_DBW_Override_Clear"
  Throttle_DBW_Enable/1 -> Throttle_Command/5  "Throttle_DBW_Enable"
  Throttle_Reserved1/1 -> Throttle_Command/8  "Throttle_Reserved1"
  Throttle_Pedal_Cmd_Type/1 -> Throttle_Command/4  "Throttle_Pedal_Cmd_Type"
  Throttle_Pedal_Cmd_Pct/1 -> Throttle_Command/3  "Throttle_Pedal_Cmd_Pct"
  zero/1 -> Throttle_Command/1  "Throttle_Pedal_Cmd_None"
  Throttle_Pedal_Cmd_Raw/1 -> Throttle_Command/2  "Throttle_Pedal_Cmd_Raw"

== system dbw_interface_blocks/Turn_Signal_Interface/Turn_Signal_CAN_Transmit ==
  Turn_Signal_Cmd : Inport
  Data Type Conversion : DataTypeConversion  OutDataTypeStr=uint8
  TurnSignal_Command : rtican/RTICAN Transmit (TX)   Reserved1=[]  Reserved2=[]  Reserved3=[]  Reserved4=[]  SfcnMessage=[]  Msg_Struct=[]  BoardTypeNo=[]  BoardNo=[]  ChannelNo=[]  Parameters=[]  DialogFcn=[]  UnitName=[]  Revision=[]  UnitValues=[]  DSProperties=struct('RTI',struct('Version',uint32(5),'BlockType',struct('isSLSource',uint8(1),'isSLSink',uint8(1),'isHWSource',uint8(0),'isHWSink',uint8(0),'isSetup',uint8(0),'isInline',uint8(1),'isNonInline',uint8(0),'isInterrupt',uint8(0),'isChannelwise',uint8(0)),'IOBoardType','RTICAN','UnitType','MESSAGE','Identifier','TX','DialogType','MSVC','BlockSet','RTICAN','SlaveProcessor','CAN'))  RTIBlockInterface=struct('InputPortsWidth',int32(1),'InputPortsActive',1,'InputPortsName',{{'TRNCMD'}},'InputPortsDataType',{{'SS_UINT8'}},'OutputPortsWidth',int32(0),'OutputPortsActive',0,'OutputPortsName',{{''}},'DialogFcn','rtican_message_interface_gui','BlockDisplay',{{'','center'}},'IconTransparency','on','InitLevel',3,'BlockName',struct('Token',{{'TurnSignal_Command'}}),'SampleTime',{{0.1}},'TriggerPort',{{'n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  RTIBlockParameters=struct('BoardTypeNo',{{1,'OFF',[]}},'BoardNo',{{1,'ON',[1 16]}},'ChannelNo',{{1,'ON',[1 2]}},'Parameters',{{struct('DataFileSupport',struct('DataFileSelectedMaster',1,'DataFileSelectedLocal',1,'DataFileName','c:\users\dataspeed\documents\matlab\dataspeed_dbw_dspace_simulink_library\lib\dataspeedbywire_19_oct_2017.dbc|','DataFileDate',['11-Jul-2018 12:27:42'],'SelectedFile','dataspeedbywire.dbc','I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  RTISFcnParameters=struct('SFcnRTICANMessage','struct','TLCFileName','char')  RTIBlockParaDefault=struct('BoardTypeNo',4302,'BoardNo',1,'ChannelNo',1,'Parameters',struct('DataFileSupport',struct('DataFileSelectedMaster',0,'DataFileSelectedLocal',0,'DataFileName','','DataFileDate','','SelectedFile',['<no file selected>']),'Options',struct('StatusSelected',1,'TimeSelected',1,'DeltaTimeSelected',1,'DelayTimeSelected',1,'DelayTimeTXCommandSelected',0,'EncodeSetUnusedBitsToOne',0,'EnableMsgLoopback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
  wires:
  Data Type Conversion/1 -> TurnSignal_Command/1
  Turn_Signal_Cmd/1 -> Data Type Conversion/1  "Turn_Signal_Cmd"
